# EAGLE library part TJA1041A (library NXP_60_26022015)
High-speed CAN transceiver The TJA1041A provides an advanced interface between the protocol controller and the physical bus in a Controller Area Network (CAN) node. The TJA1041A is primarily intended for automotive high-speed CAN applications (up to 1 Mbit/s). The transceiver provides differential transmit capability to the bus and differential receive capability to the CAN controller. The TJA1041A is fully compatible to the ISO 11898 standard, and offers excellent ElectroMagnetic Compatibility (EMC) performance, very low power consumption, and passive behavior when supply voltage is off. The advanced features include: Low-power management, supporting local and remote wake-up with wake-up source recognition and the capability to control the power supply in the rest of the node Several protection and diagnosis functions including short circuits of the bus lines and ﬁrst battery connection Automatic adaptation of the I/O-levels, in line with the supply voltage of the controller AAL Eindhoven MK
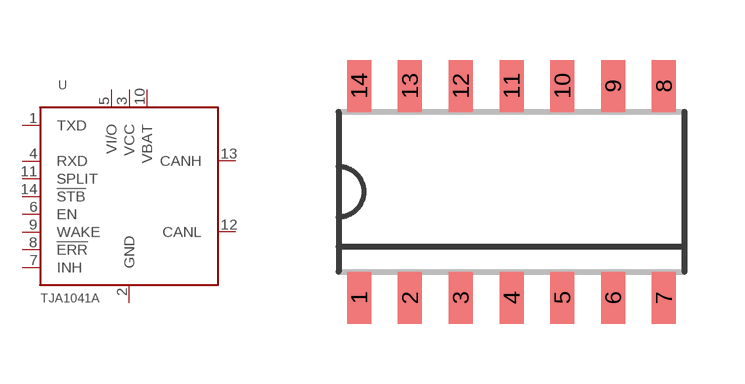
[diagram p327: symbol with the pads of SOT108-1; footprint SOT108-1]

Designator prefix U

## TJA1041AT  [SOT108-1]
1  TXD  out
2  GND  pwr
3  VCC  pwr
4  RXD
5  VI/O  pwr
6  EN  in
7  INH  in
8  !ERR  out
9  WAKE  in
10  VBAT  pwr
11  SPLIT  pwr
12  CANL
13  CANH
14  !STB  in

## Footprint SOT108-1 (pad centres in mm)
SOT108-1 SO14: plastic small outline package; 14 leads; body width 3.9 mm; body thickness 1.47 mm JEDEC: MS-012 IEC: --
smd 0.6 x 1.3: 1 -3.81,-2.65; 2 -2.54,-2.65; 3 -1.27,-2.65; 4 0,-2.65; 5 1.27,-2.65; 6 2.54,-2.65; 7 3.81,-2.65; 8 3.81,2.65; 9 2.54,2.65; 10 1.27,2.65; 11 0,2.65; 12 -1.27,2.65; 13 -2.54,2.65; 14 -3.81,2.65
